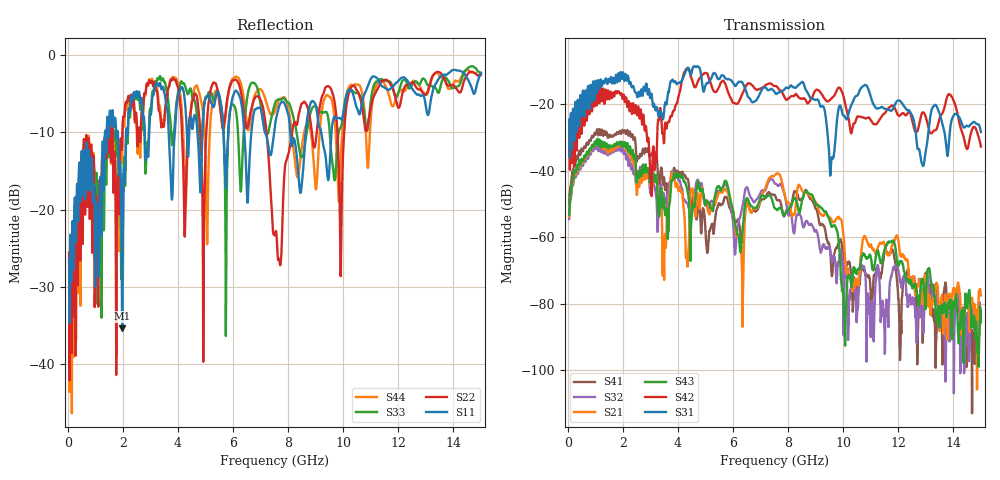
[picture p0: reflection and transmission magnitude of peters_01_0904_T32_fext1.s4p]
# MHZ S RI R 50.00
! FREQ  S11  S12  S13  S14
!  S21  S22  S23  S24
!  S31  S32  S33  S34
!  S41  S42  S43  S44
!  REAL  IMAG  REAL  IMAG  REAL  IMAG  REAL  IMAG
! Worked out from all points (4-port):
!   1496 points, 50 MHz to 15 GHz, reference 50 ohm
!   strongest paths, dB at 50 MHz, 3.79 GHz, 7.53 GHz, 11.27 GHz, 15 GHz:
!     S31: -24.8, -12.8, -16.7, -21.3, -28.4
!     S42: -24.8, -23.3, -14.6, -25.3, -32.8
!     S43: -53.3, -42.9, -51.4, -64.3, -85.4
!     S21: -53.8, -40.6, -41.3, -62.7, -77.6
!     S32: -54.6, -40.3, -44.0, -68.8, -84.2
!     S41: -50.3, -40.4, -47.5, -69.5, -82.9
!   lowest |S11| = -35.3 dB at 1.98 GHz (marker M1), VSWR 1.03, Z = 51.6 + j0.56 ohm
!   |S11| at or under -10 dB: start of sweep to 1.354 GHz; 8.078 GHz to 8.638 GHz (559.9 MHz wide, 6.7 % of centre); 9.203 GHz to 9.576 GHz (372.9 MHz wide, 3.97 % of centre)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
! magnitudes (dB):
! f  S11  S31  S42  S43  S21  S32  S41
! 50 MHz  -26.5  -24.8  -24.8  -53.3  -53.8  -54.6  -50.3
! 1.98 GHz  -35.3  -12.0  -18.3  -31.4  -31.3  -33.0  -27.8
! 3.5 GHz  -4.9  -21.9  -31.6  -49.1  -72.9  -47.4  -42.4
! 3.81 GHz  -17.4  -12.7  -22.5  -43.0  -41.1  -40.9  -40.6
! 7.63 GHz  -7.2  -16.7  -15.1  -51.8  -40.9  -44.6  -49.0
! 10.22 GHz  -4.5  -22.1  -25.4  -71.8  -71.7  -79.0  -67.5
! 15 GHz  -2.4  -28.4  -32.8  -85.4  -77.6  -84.2  -82.9
